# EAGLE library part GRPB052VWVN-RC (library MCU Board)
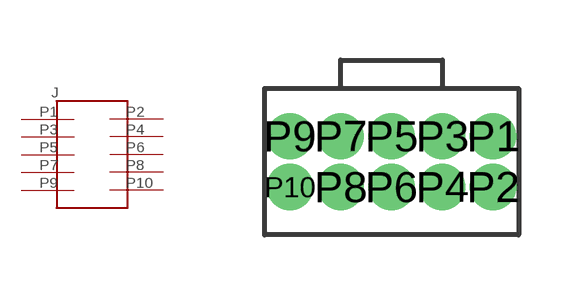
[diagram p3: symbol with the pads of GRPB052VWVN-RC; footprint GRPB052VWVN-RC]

Designator prefix J

## GRPB052VWVN-RC  [GRPB052VWVN-RC]
P1  P$1
P2  P$2
P3  P$3
P4  P$4
P5  P$5
P6  P$6
P7  P$7
P8  P$8
P9  P$9
P10  P$10

## Footprint GRPB052VWVN-RC (pad centres in mm)
drill 0.65 pad 0.9: P1 2.54,0.635; P2 2.54,-0.635; P3 1.27,0.635; P4 1.27,-0.635; P5 0,0.635; P6 0,-0.635; P7 -1.27,0.635; P8 -1.27,-0.635; P9 -2.54,0.635; P10 -2.54,-0.635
